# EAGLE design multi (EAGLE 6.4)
Assembly variants: VUSB, FT232
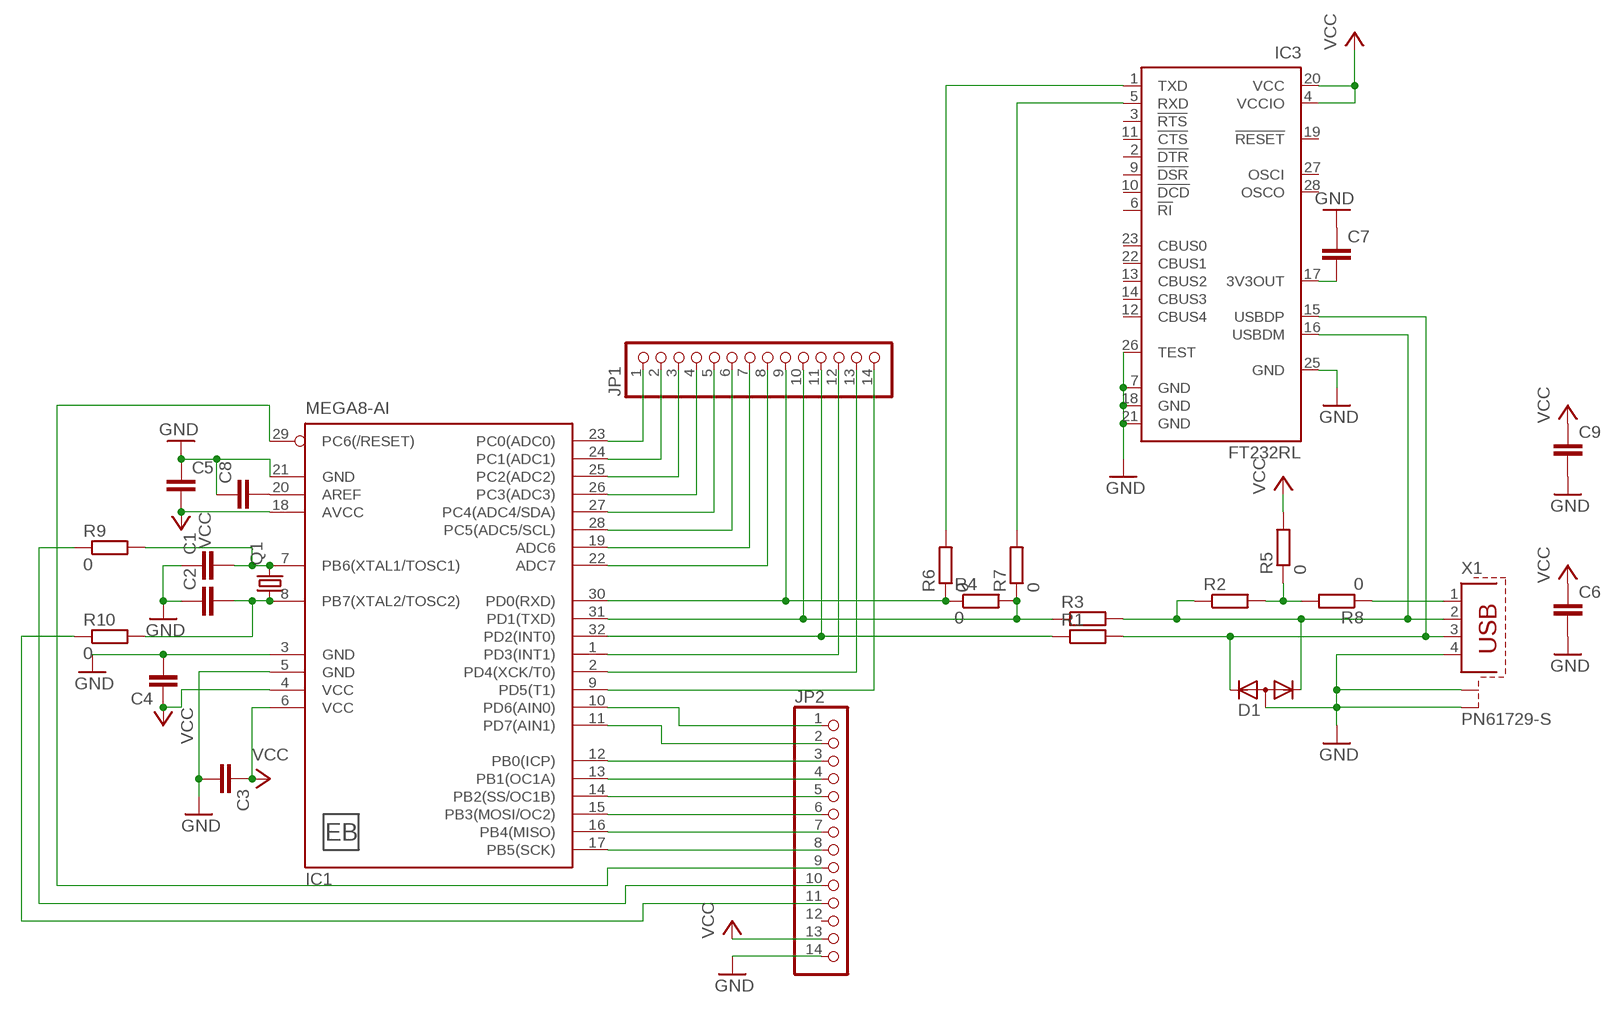
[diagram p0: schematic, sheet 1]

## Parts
C1  C-EUC0805  [C0805]  (variant VUSB: 18p)  (variant FT232: 18p)
C2  C-EUC0805  [C0805]  (variant VUSB: 18p)  (variant FT232: 18p)
C3  C-EUC0805  [C0805]  (variant VUSB: 100n)  (variant FT232: 100n)
C4  C-EUC0805  [C0805]  (variant VUSB: 100n)  (variant FT232: 100n)
C5  C-EUC0805  [C0805]  (variant VUSB: 100n)  (variant FT232: 100n)
C6  C-EUC0805  [C0805]  (variant VUSB: 100n)  (variant FT232: 100n)
C7  C-EUC0805  [C0805]  (not fitted in variant VUSB)
C8  C-EUC0805  [C0805]  (variant VUSB: 100n)  (variant FT232: 100n)
C9  C-EUC0805  [C0805]  (variant VUSB: 100n)  (variant FT232: 100n)
D1  DIODE-2CA|ACSOT23  [SOT23]  (not fitted in variant FT232)
IC1  MEGA8-AI  [TQFP32-08]
IC3  FT232RL  [SSOP28]  (not fitted in variant VUSB)
JP1  PINHD-1X14  [1X14]
JP2  PINHD-1X14  [1X14]
Q1  CRYSTALHC49S  [HC49/S]
R1  R-EU_R0805  [R0805]  (variant VUSB: 68)  (not fitted in variant FT232)
R2  R-EU_R0805  [R0805]  (variant VUSB: 1k5)  (not fitted in variant FT232)
R3  R-EU_R0805  [R0805]  (variant VUSB: 68)  (not fitted in variant FT232)
R4  0  R-EU_R0805  [R0805]  (not fitted in variant FT232)
R5  0  R-EU_R0805  [R0805]
R6  0  R-EU_R0805  [R0805]  (not fitted in variant VUSB)
R7  0  R-EU_R0805  [R0805]  (not fitted in variant VUSB)
R8  0  R-EU_R0805  [R0805]
R9  0  R-EU_R0805  [R0805]  (not fitted in variant VUSB)  (not fitted in variant FT232)
R10  0  R-EU_R0805  [R0805]  (not fitted in variant VUSB)  (not fitted in variant FT232)
U$1  EB  [EB]
X1  PN61729-S  [PN61729-S]

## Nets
GND: C1.1 C2.1 C3.2 C4.2 C5.1 C6.2 C7.1 C8.1 C9.2 D1.3(A) IC1.3(GND) IC1.5(GND) IC1.21(GND) IC3.7(GND) IC3.18(GND) IC3.21(GND) IC3.25(GND) IC3.26(TEST) JP2.14 X1.4 X1.S1 X1.S2
N$1: JP2.10 R9.1
N$2: JP2.11 R10.1
N$3: IC1.31(PD1(TXD)) JP1.10 R3.1 R4.2 R7.1
N$4: D1.1(K1) IC3.16(USBDM) R2.1 R3.2 X1.2
N$5: R2.2 R5.1 R8.2
N$6: D1.2(K2) IC3.15(USBDP) R1.2 X1.3
N$7: IC1.32(PD2(INT0)) JP1.11 R1.1
N$8: IC1.30(PD0(RXD)) JP1.9 R4.1 R6.1
N$9: R8.1 X1.1
N$10: IC1.23(PC0(ADC0)) JP1.1
N$11: C7.2 IC3.17(3V3OUT)
N$12: IC3.1(TXD) R6.2
N$13: IC3.5(RXD) R7.2
N$14: IC1.24(PC1(ADC1)) JP1.2
N$15: IC1.25(PC2(ADC2)) JP1.3
N$16: IC1.26(PC3(ADC3)) JP1.4
N$17: IC1.27(PC4(ADC4/SDA)) JP1.5
N$18: IC1.28(PC5(ADC5/SCL)) JP1.6
N$19: IC1.19(ADC6) JP1.7
N$20: IC1.22(ADC7) JP1.8
N$21: IC1.1(PD3(INT1)) JP1.12
N$22: IC1.2(PD4(XCK/T0)) JP1.13
N$23: IC1.9(PD5(T1)) JP1.14
N$24: IC1.10(PD6(AIN0)) JP2.1
N$25: IC1.11(PD7(AIN1)) JP2.2
N$26: IC1.12(PB0(ICP)) JP2.3
N$27: IC1.13(PB1(OC1A)) JP2.4
N$28: IC1.14(PB2(SS/OC1B)) JP2.5
N$29: IC1.15(PB3(MOSI/OC2)) JP2.6
N$30: IC1.16(PB4(MISO)) JP2.7
N$31: IC1.17(PB5(SCK)) JP2.8
N$32: C1.2 IC1.7(PB6(XTAL1/TOSC1)) Q1.2 R9.2
N$33: IC1.29(PC6(/RESET)) JP2.9
N$34: C2.2 IC1.8(PB7(XTAL2/TOSC2)) Q1.1 R10.2
N$35: C8.2 IC1.20(AREF)
VCC: C3.1 C4.1 C5.2 C6.1 C9.1 IC1.4(VCC) IC1.6(VCC) IC1.18(AVCC) IC3.4(VCCIO) IC3.20(VCC) JP2.13 R5.2
Unconnected: IC3.2(!DTR) IC3.3(!RTS) IC3.6(!RI) IC3.9(!DSR) IC3.10(!DCD) IC3.11(!CTS) IC3.12(CBUS4) IC3.13(CBUS2) IC3.14(CBUS3) IC3.19(!RESET) IC3.22(CBUS1) IC3.23(CBUS0) IC3.27(OSCI) IC3.28(OSCO) JP2.12

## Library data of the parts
C1-C9 = rcl:C-EU: CAPACITOR, European symbol
D1 = diode:DIODE-2CA|AC: Dual DIODE Cathode-Anode|Anode-Cathode
IC1 = atmel:MEGA8: MICROCONTROLLER 8 Kbytes FLASH, 1 kbytes SRAM, 512 bytes EEPROM, USART, 6-channel 10 bit ADC, 2-channel 8 bit ADC Pin compatible with Atmega48, ATMega88, ATMega168 Source: avr.lbr; MPN: ATMEGA8-16AU; OC_FARNELL: 9171371; OC_NEWARK: 73M8863
IC3 = ftdichip:FT232R: Source: http://www.ftdichip.com/Documents/DataSheets/DS_FT232R_v104.pdf; MPN: FT232RL; OC_FARNELL: 1146032; OC_NEWARK: 91K9918
JP1 JP2 = pinhead:PINHD-1X14: PIN HEADER
Q1 = crystal:CRYSTAL: CRYSTAL; OC_FARNELL: 1667008; OC_NEWARK: unknown
R1-R10 = rcl:R-EU_: RESISTOR, European symbol
U$1 = Jakob:EB
X1 = con-berg:PN61729-S: BERG USB connector; OC_FARNELL: unknown; OC_NEWARK: unknown

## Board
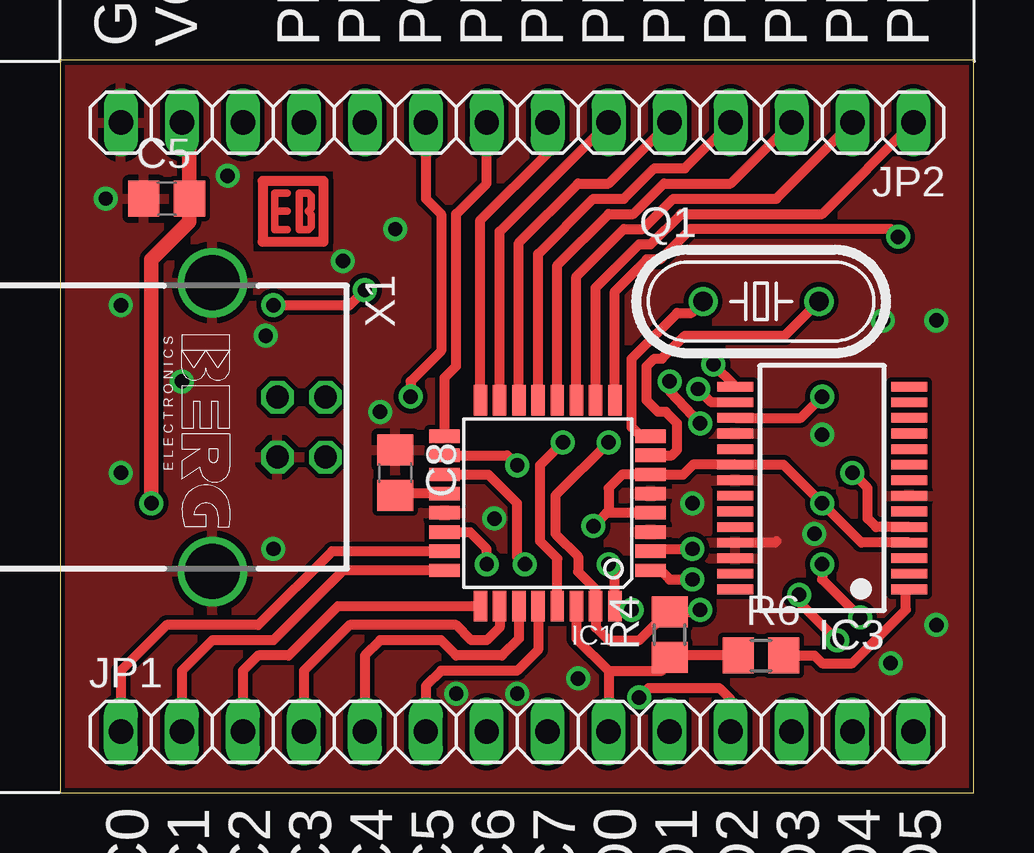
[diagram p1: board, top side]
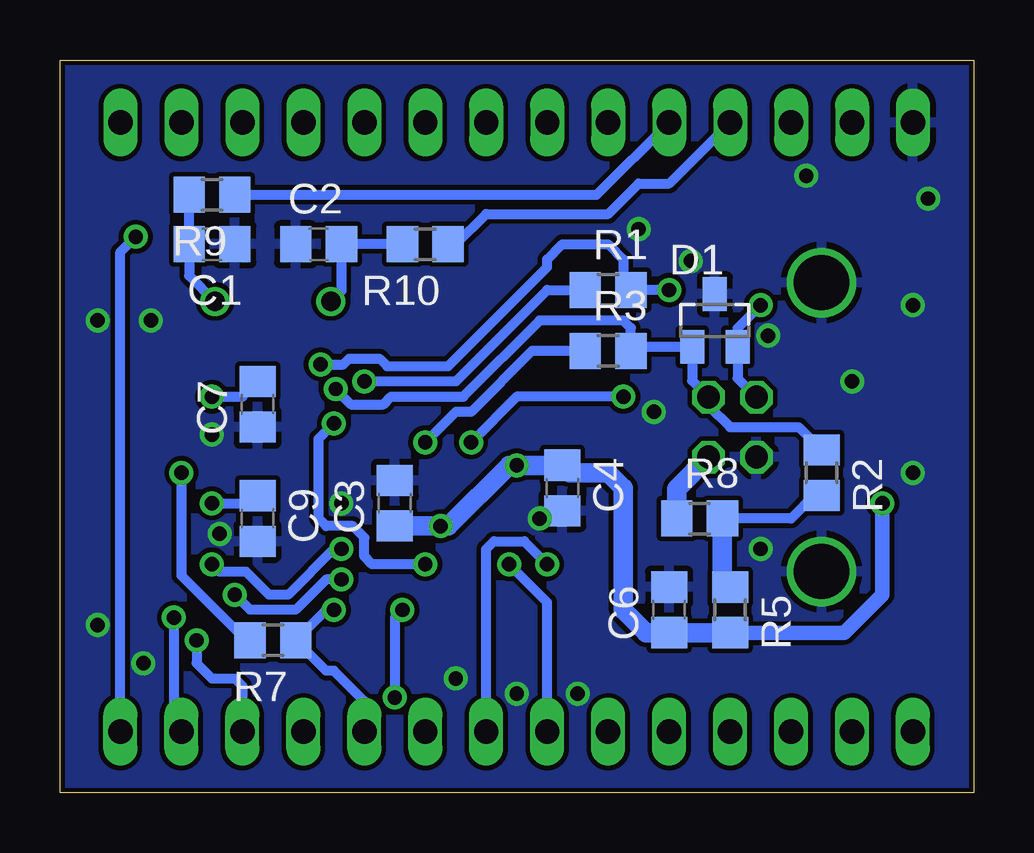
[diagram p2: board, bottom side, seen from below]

Size 38.08 x 30.55 mm. Coordinates in mm from the lower left corner, seen from the top.
Outline: 0,0 38.08,0 38.08,30.55 0,30.55 0,0
Copper layers (1*16): Top 0.035mm / dielectric 1.5mm / Bottom 0.035mm
Design rules "default": minimum track width 0.2mm, minimum drill 0.5mm, track to track 0.2mm, track to pad 0.2mm, pad to pad 0.15mm, via to via 0.2mm, smd to smd 0mil, copper to edge 0.2mm, drill to drill 0.2mm, minimum pad ring 0.2mm, minimum via ring 0.2mm, stop-mask expansion 0.1mm, vias tented up to drill 0mil, thermal gap 10mil

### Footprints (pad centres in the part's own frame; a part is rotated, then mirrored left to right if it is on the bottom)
C0805 = smd 1.3 x 1.5: 1 -0.95,0; 2 0.95,0
SOT23 = smd 1 x 1.4: 1 -0.95,-1.1; 2 0.95,-1.1; 3 0,1.1
TQFP32-08 = smd 1.27 x 0.559: 1 -4.293,2.8; 2 -4.293,2; 3 -4.293,1.2; 4 -4.293,0.4; 5 -4.293,-0.4; 6 -4.293,-1.2; 7 -4.293,-2; 8 -4.293,-2.8; 17 4.293,-2.8; 18 4.293,-2; 19 4.293,-1.2; 20 4.293,-0.4; 21 4.293,0.4; 22 4.293,1.2; 23 4.293,2; 24 4.293,2.8 | smd 0.559 x 1.27: 9 -2.8,-4.293; 10 -2,-4.293; 11 -1.2,-4.293; 12 -0.4,-4.293; 13 0.4,-4.293; 14 1.2,-4.293; 15 2,-4.293; 16 2.8,-4.293; 25 2.8,4.293; 26 2,4.293; 27 1.2,4.293; 28 0.4,4.293; 29 -0.4,4.293; 30 -1.2,4.293; 31 -2,4.293; 32 -2.8,4.293
SSOP28 = smd 0.4 x 1.5: 1 -4.225,-3.625; 2 -3.575,-3.625; 3 -2.925,-3.625; 4 -2.275,-3.625; 5 -1.625,-3.625; 6 -0.975,-3.625; 7 -0.325,-3.625; 8 0.325,-3.625; 9 0.975,-3.625; 10 1.625,-3.625; 11 2.275,-3.625; 12 2.925,-3.625; 13 3.575,-3.625; 14 4.225,-3.625; 15 4.225,3.625; 16 3.575,3.625; 17 2.925,3.625; 18 2.275,3.625; 19 1.625,3.625; 20 0.975,3.625; 21 0.325,3.625; 22 -0.325,3.625; 23 -0.975,3.625; 24 -1.625,3.625; 25 -2.275,3.625; 26 -2.925,3.625; 27 -3.575,3.625; 28 -4.225,3.625
1X14 = drill 1.016 long: 1 -16.51,0; 2 -13.97,0; 3 -11.43,0; 4 -8.89,0; 5 -6.35,0; 6 -3.81,0; 7 -1.27,0; 8 1.27,0; 9 3.81,0; 10 6.35,0; 11 8.89,0; 12 11.43,0; 13 13.97,0; 14 16.51,0
HC49/S = drill 0.813: 1 -2.413,0; 2 2.413,0
R0805 = smd 1.3 x 1.5: 1 -0.95,0; 2 0.95,0
PN61729-S = drill 0.95 octagon: 1 1.25,4.71; 2 -1.25,4.71; 3 -1.25,2.71; 4 1.25,2.71 | drill 2.3 pad 2.9: S1 -6.02,0; S2 6.02,0

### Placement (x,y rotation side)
C1  31.75,22.86 180 bottom
C2  27.3,22.86 0 bottom
C3  24.13,12.06 90 bottom
C4  17.14,12.7 270 bottom
C5  4.45,24.77 0 top
C6  12.7,7.62 90 bottom
C7  29.84,16.19 90 bottom
C8  13.97,13.34 270 top
C9  29.84,11.43 270 bottom
D1  10.79,19.68 0 bottom
IC1  20.32,12.06 180 top
IC3  31.75,12.7 90 top
JP1  19.05,2.54 0 top
JP2  19.05,27.94 180 top
Q1  29.21,20.48 0 top
R1  15.24,20.95 0 bottom
R2  6.35,13.34 270 bottom
R3  15.24,18.41 0 bottom
R4  25.4,6.59 90 top
R5  10.16,7.62 270 bottom
R6  29.21,5.71 0 top
R7  29.21,6.35 180 bottom
R8  11.43,11.43 0 bottom
R9  31.75,24.92 180 bottom
R10  22.86,22.86 180 bottom
U$1  9.72,24.23 0 top
X1  6.35,15.24 270 top

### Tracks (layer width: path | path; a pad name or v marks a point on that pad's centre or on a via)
GND  (via drill 0.6)
  Top 0.406: IC3.25 29.79,10.43 C9.2
  other vias: 31.43,10.79 31.75,14.92 34.29,19.68 36.51,19.68 36.51,6.99 34.61,5.4 21.59,4.76 19.05,4.13 18.1,11.43 16.51,4.13 8.89,10.16 8.57,19.05 2.54,13.34 2.54,20.32 6.99,25.72 5.08,17.14 11.79,22.17 13.97,23.5 1.91,24.77 26.35,12.06 13.34,15.88
  pour Bottom: 0,30.48 0,0 38.1,0 38.1,30.48
  pour Top: 0,30.48 0,0 38.1,0 38.1,30.48
N$1
  Bottom 0.406: R9.1 15.72,24.92 JP2.10
N$2
  Bottom 0.406: R10.1 21.59,22.86 20.32,24.13 15.24,24.13 13.97,25.4 12.7,25.4 JP2.11
N$3  (via drill 0.6)
  Top 0.406: v26.67,7.62 26.51,7.54 R4.2 25.24,7.14 24.92,7.14 24.13,6.35 22.86,6.35 22.32,6.89 IC1.31 22.32,8.48 21.59,9.21 21.59,9.84 20.64,10.79 20.64,12.38 v22.86,14.61
  Bottom 0.406: v26.67,7.62 26.99,7.62 R7.1 26.99,5.08 26.67,5.08 25.4,3.81 JP1.10 | R3.1 18.41,18.41 20.95,15.88 21.59,15.88 v22.86,14.61
N$4  (via drill 0.6)
  Top 0.406: IC3.16 27.14,16.27 v26.59,16.83
  Bottom 0.406: v26.59,16.83 25.96,16.19 24.61,16.19 24.29,16.51 21.27,16.51 18.1,19.68 14.61,19.68 14.29,19.37 R3.2 14.12,18.59 D1.1 11.74,17.18 X1.2 11.06,16.14 10.16,15.24 7.3,15.24 R2.1
N$5
  Bottom 0.406: R2.2 6.67,12.38 7.62,11.43 R8.2
  Bottom 0.813: R8.2 10.48,8.89 R5.1
N$6  (via drill 0.6)
  Top 0.406: v8.89,20.32 12.06,20.32 v12.7,20.95 | IC3.15 28.12,16.96 v27.23,17.86
  Bottom 0.406: X1.3 9.85,17.27 D1.2 9.85,19.36 v8.89,20.32 | v12.7,20.95 R1.2 14.61,21.27 14.61,22.23 15.24,22.86 17.14,22.86 17.78,22.23 17.78,21.91 21.91,17.78 24.45,17.78 24.77,18.1 26.04,18.1 26.27,17.86 v27.23,17.86
N$7  (via drill 0.6)
  Top 0.406: v23.81,7.62 23.27,7.62 IC1.32 23.12,9.27 v22.86,9.53 | v25.4,17.14 25.4,16.75 v26.67,15.4 | v24.13,3.97 24.53,4.37 27.46,4.37 27.94,3.89 JP1.11
  Bottom 0.406: v23.81,7.62 24.13,7.3 v24.13,3.97 | v22.86,9.53 25.08,9.53 25.4,9.84 25.4,10.64 25.88,11.11 26.99,11.11 27.3,11.43 27.3,14.76 v26.67,15.4 | R1.1 17.78,20.95 21.59,17.14 v25.4,17.14
N$8
  Top 0.406: R6.1 25.71,5.71 R4.1 25.08,5.08 22.86,5.08 | IC1.30 21.52,6.42 22.86,5.08 | 22.86,5.08 JP1.9
N$9
  Bottom 0.813: R8.1 12.38,12.67 X1.1
N$10
  Top 0.406: IC1.23 11.34,10.06 8.26,6.99 4.45,6.99 2.54,5.08 JP1.1
N$11  (via drill 0.6)
  Top 0.406: IC3.17 30.86,15.62 v31.75,16.51
  Bottom 0.406: v31.75,16.51 30.48,16.51 C7.2
N$12
  Top 0.406: R6.2 31.43,5.71 31.75,5.4 33.02,5.4 35.24,7.62 35.24,8.34 IC3.1
N$13  (via drill 0.6)
  Top 0.406: IC3.5 34.01,11.07 33.66,11.43 33.66,12.7 v33.02,13.34
  Bottom 0.406: v33.02,13.34 33.02,9.05 30.32,6.35 R7.2
N$14
  Top 0.406: IC1.24 11.8,9.27 8.89,6.35 6.35,6.35 5.08,5.08 JP1.2
N$15
  Top 0.406: IC1.25 11.58,7.77 9.53,5.71 8.26,5.71 7.62,5.08 JP1.3
N$16
  Top 0.406: IC1.26 18.32,6.89 17.78,6.35 17.14,6.35 16.51,6.99 12.06,6.99 10.16,5.08 JP1.4
N$17
  Top 0.406: IC1.27 19.12,6.42 18.41,5.71 16.51,5.71 15.88,6.35 13.34,6.35 12.7,5.71 JP1.5
N$18
  Top 0.406: IC1.28 19.92,5.95 19.05,5.08 15.88,5.08 15.24,4.45 JP1.6
N$19  (via drill 0.6)
  Top 0.406: v19.37,9.53 19.05,9.84 19.05,12.06 17.85,13.27 IC1.19
  Bottom 0.406: JP1.7 17.78,7.94 v19.37,9.53
N$20  (via drill 0.6)
  Top 0.406: v17.78,9.53 17.78,10.16 17.07,10.87 IC1.22
  Bottom 0.406: JP1.8 20.32,10.16 20,10.48 18.73,10.48 v17.78,9.53
N$21  (via drill 0.6)
  Top 0.406: IC1.1 25.02,9.27 25.4,8.89 v26.35,8.89 | v30.8,8.26 30.8,7.94 v32.38,6.35
  Bottom 0.406: v26.35,8.89 26.99,8.89 28.26,7.62 30.16,7.62 v30.8,8.26 | v32.38,6.35 32.38,5.4 31.75,4.76 30.8,4.76 30.48,4.45 JP1.12
N$22  (via drill 0.6)
  Top 0.406: IC1.2 24.99,10.06 25.08,10.16 v26.35,10.16 | v31.75,9.53 31.75,8.89 v33.34,7.3
  Bottom 0.406: v26.35,10.16 26.67,10.16 28.57,8.26 29.37,8.26 30.32,9.21 31.43,9.21 v31.75,9.53 | v33.34,7.3 33.34,2.86 JP1.13
N$23  (via drill 0.6)
  Top 0.406: v34.92,23.18 34.61,23.5 26.27,23.5 25,22.23 24.45,22.23 23.12,20.9 IC1.9
  Bottom 0.406: JP1.14 35.56,22.54 v34.92,23.18
N$24
  Top 0.406: IC1.10 22.32,21.05 24.13,22.86 24.61,22.86 25.88,24.13 31.75,24.13 JP2.1
N$25
  Top 0.406: IC1.11 21.52,21.52 23.5,23.5 24.29,23.5 25.56,24.77 29.84,24.77 JP2.2
N$26
  Top 0.406: IC1.12 20.72,21.99 22.86,24.13 23.89,24.13 25.16,25.4 27.94,25.4 JP2.3
N$27
  Top 0.406: IC1.13 19.92,22.46 22.23,24.77 23.5,24.77 24.77,26.04 26.04,26.04 JP2.4
N$28
  Top 0.406: IC1.14 19.12,22.93 21.59,25.4 22.86,25.4 JP2.5
N$29
  Top 0.406: IC1.15 18.32,23.4 JP2.6
N$30
  Top 0.406: IC1.16 17.52,23.87 20.32,26.67 JP2.7
N$31
  Top 0.406: IC1.17 16.03,17.3 16.51,17.78 16.51,24.13 17.78,25.4 JP2.8
N$32
  Top 0.406: IC1.7 25.5,14.06 25.72,14.29 25.72,15.4 25.24,15.88 24.92,15.88 24.45,16.35 24.45,17.78 24.77,18.1 25.08,18.1 26.04,19.05 30.19,19.05 Q1.2
  Bottom 0.406: Q1.2 32.7,21.56 C1.2 R9.2
N$33  (via drill 0.6)
  Top 0.406: JP2.9 15.24,24.77 15.88,24.13 15.88,18.41 14.61,17.14 v14.61,16.51 | IC1.29 20.72,9.76 20,10.48 20,13.65 v20.95,14.61
  Bottom 0.406: v14.61,16.51 19.05,16.51 v20.95,14.61
N$34
  Top 0.406: IC1.8 24.19,14.87 23.81,15.24 23.81,18.1 25.72,20 26.32,20 Q1.1
  Bottom 0.406: Q1.1 26.36,20.92 C2.2 R10.2
N$35
  Top 0.406: IC1.20 14.05,12.46 C8.2
VCC  (via drill 0.6)
  Top 0.406: IC1.18 18.64,14.06 v19.05,13.65 | IC1.4 22.77,11.66 | 22.77,11.66 v22.23,11.12 | 22.77,11.66 22.86,11.75 22.86,12.7 23.43,13.27 IC1.6 25.96,13.27 26.38,13.68 IC3.20 30.14,13.68 v31.75,12.06 33.39,10.43 IC3.4
  Top 0.61: JP2.13 5.39,27.62 C5.2 5.39,23.81 3.81,22.23 v3.81,12.06
  Bottom 0.406: v31.75,12.06 30.16,12.06 C9.1
  Bottom 0.61: v3.81,12.06 3.81,8.26 5.39,6.67 R5.2
  Bottom 0.813: R5.2 C6.1 13.65,6.67 14.61,7.62 14.61,12.7 15.24,13.34 16.83,13.34 C4.1 v19.05,13.65 19.37,13.65 21.91,11.12 v22.23,11.12 C3.1

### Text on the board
tNames: XTAL2/TOSC2 | XTAL1/TOSC1 | RESET | SCK | MISO | MOSI/OC2 | SS/OC1B | OC1A | ICP | AIN1 | AIN0 | GND | VCC | PB7 | PB6 | PC6 | PB5 | PB4 | PB3 | PB2 | PB1 | PB0 | PD7 | PD6 | PC0 | PC1 | PC2 | PC3 | PC4 | PC5 | ADC6 | ADC7 | PD0 | PD1 | PD2 | PD3 | PD4 | PD5 | RXD | TXD | INT0 | INT1 | XCK/T0 | T1 | ADC 0 - 7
